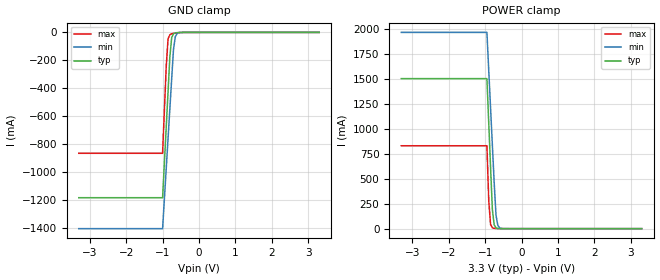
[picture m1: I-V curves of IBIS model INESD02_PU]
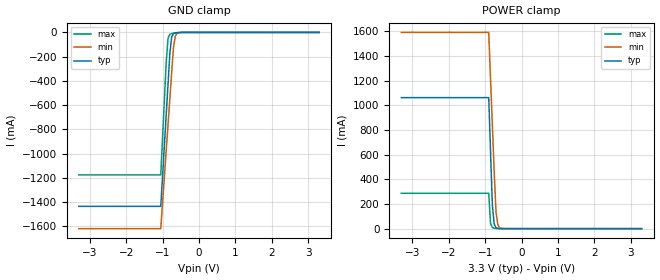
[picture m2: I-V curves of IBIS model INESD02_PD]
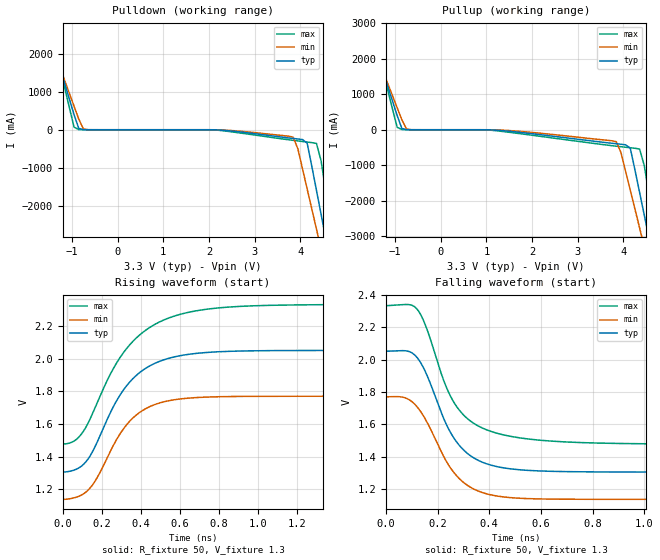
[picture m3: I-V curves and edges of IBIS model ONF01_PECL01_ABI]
|   This file is an IBIS representation of the   |
|   Integrated Devices Technology, Inc.   |
|   ICS843003I-01   |
|   FEMTOCLOCKS CRYSTAL-TO-3.3V/2.5V LVPECL FREQUENCY SYNTHESIZER   |
[IBIS Ver]   4.1
[File name]   843003i_01_3v3.ibs
[File Rev]   1.0
[Date]   24 Dec 2008 | Last modified
|   24 Dec 2008 | Generated
[Source]   Originated at Integrated Devices Technology, Inc.
[Disclaimer]
IDT hereby grants the user of this IBIS model a non-exclusive,
nontransferable license to use this IBIS model under the following terms.
Before using this IBIS model, the user should read this license.
If the user does not accept these terms,  the IBIS model should be
returned to IDT within 30 days.
   The user is granted this license only to use the IBIS model and
is not granted rights to sell, load, rent, lease or license the IBIS
model in whole or in part, or in modified form to anyone other than
user. User may modify the IBIS model to suit its specific
applications but rights to derivative works and such modifications
shall belong to IDT.
   This IBIS model is provided on an "AS IS" basis and IDT makes
absolutely no warranty with respect to the information contained
herein. IDT DISCLAIMS AND CUSTOMER WAIVES ALL WARRANTIES, EXPRESS
OR IMPLIED, INCLUDING WARRANTIES OF MERCHANTABILITY OR FITNESS FOR
A PARTICULAR PURPOSE. The entire risk as to quality and performance
is with the Customer. ACCORDINGLY, IN NO EVENT SHALL THE COMPANY BE
LIABLE FOR ANY DAMAGES, WHETHER IN CONTRACT OR TORT,INCLUDING ANY
LOST PROFITS OR OTHER INCIDENTAL, CONSEQUENTIAL, EXEMPLARY, OR
PUNITIVE DAMAGES ARISING OUT OF THE USE OR APPLICATION OF THE IBIS
model provided in this package. Further, IDT reserves the right to
make changes without notice to any product herein to improve
reliability, function, or design. IDT does not convey any license
under patent rights or any other intellectual property rights,
including those of third parties.
   IDT is not obligated to provide maintenance or support
for the licensed IBIS model.
[Copyright]   Copyright 2004 byIntegrated Devices Technology, Inc.
[Component]   ICS843003I-01
[Manufacturer] Integrated Devices Technology, Inc.
[Package]
|TSSOP 24 Lead
|   typ   min   max
R_pkg   60.65m   52.4m   68.9m
L_pkg   1.989nH   1.431nH   2.547nH
C_pkg   0.314pF   0.254pF   0.374pF
[Pin]   signal_name   model_name   R_pin   L_pin   C_pin
1   DIV_SELB0   INESD02_PU   68.9m   2.547n   0.374p
2   VCO_SEL   INESD02_PU   65.6m   2.323n   0.350p
3   MR   INESD02_PD   62.3m   2.100n   0.326p
4   VCCO_A   POWER   59.0m   1.877n   0.302p
5   QA0   ONF01_PECL01_ABI   55.7m   1.654n   0.278p
6   nQA0   ONF01_PECL01_ABI   52.4m   1.431n   0.254p
7   OEB   INESD02_PU_PECL   52.4m   1.431n   0.254p
8   OEA   INESD02_PU_PECL   55.7m   1.654n   0.278p
9   FB_DIV   INESD02_PD   59.0m   1.877n   0.302p
10   VCCA   POWER   62.3m   2.100n   0.326p
11   VCC   POWER   65.6m   2.323n   0.350p
12   DIV_SELA0   INESD02_PU   68.9m   2.547n   0.374p
13   DIV_SELA1   INESD02_PU   68.9m   2.547n   0.374p
14   VEE   GND   65.6m   2.323n   0.350p
15   XTAL_OUT   NC   62.3m   2.100n   0.326p
16   XTAL_IN   NC   59.0m   1.877n   0.302p
17   REF_CLK   INESD02_PD_PECL   55.7m   1.654n   0.278p
18   XTAL_SEL   INESD02_PU   52.4m   1.431n   0.254p
19   nQB1   ONF01_PECL01_ABI   52.4m   1.431n   0.254p
20   QB1   ONF01_PECL01_ABI   55.7m   1.654n   0.278p
21   nQB0   ONF01_PECL01_ABI   59.0m   1.877n   0.302p
22   QB0   ONF01_PECL01_ABI   62.3m   2.100n   0.326p
23   VCCO_B   POWER   65.6m   2.323n   0.350p
24   DIV_SELB1   INESD02_PU   68.9m   2.547n   0.374p
[Diff Pin]  inv_pin  vdiff tdelay_typ tdelay_min  tdelay_max
5   6   NA   0   0   0
20   19   NA   0   0   0
23   22   NA   0   0   0
| Models and submodels in the file (5): INESD02_PU (Input), INESD02_PD (Input), ONF01_PECL01_ABI (Output_ECL), INESD02_PU_PECL (Input), INESD02_PD_PECL (Input)
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[Model]   INESD02_PU
Model_type   Input
Polarity   Non-Inverting
Vinl = 0.80V
Vinh = 2.0V
|   typ   min   max
C_comp   2pF   1.5pF   2.5pF
|   typ   min   max
[Voltage range]  3.3V   3.15V   3.45V
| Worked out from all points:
|   GND clamp passes 1 mA (typ) near -0.56 V on its own axis
|   POWER clamp passes 1 mA (typ) near -0.61 V on its own axis
[GND_clamp]
|Voltage   I(typ)   I(min)   I(max)
-3.3V     -1.184A    -1.405A    -865.6mA
-1V       -1.184A    -1.405A    -865.6mA
-900mV    -678.5mA   -975.1mA   -244.1mA
-850mV    -426.2mA   -760.2mA   -46.92mA
-800mV    -174mA     -545.4mA   -16.17mA
-750mV    -37.03mA   -330.8mA   -9.981mA
-700mV    -9.767mA   -120.3mA   -7.122mA
-650mV    -3.616mA   -29.78mA   -4.922mA
-600mV    -1.7mA     -7.594mA   -3.115mA
-400mV    -123.9uA   -126uA     -173.9uA
3.3V      1.866nA    3.949uA    0A
[POWER_clamp]
|Voltage   I(typ)   I(min)   I(max)
-3.3V     1.506A     1.97A      832.1mA
-950mV    1.506A     1.97A      832.1mA
-900mV    1.063A     1.592A     287.2mA
-850mV    620.4mA    1.215A     41.77mA
-800mV    191.5mA    837.4mA    8.692mA
-750mV    37.69mA    460.1mA    3.262mA
-700mV    8.032mA    133.8mA    1.662mA
-650mV    2.005mA    32.58mA    840.1uA
-600mV    607uA      8.009mA    378.6uA
-450mV    33.11uA    139.8uA    23.88uA
3.3V      -71.13uA   -77.46uA   -62.11uA
[Model]   INESD02_PD
Model_type   Input
Polarity   Non-Inverting
Vinl = 0.80V
Vinh = 2.0V
|   typ   min   max
C_comp   2pF   1.5pF   2.5pF
|   typ   min   max
[Voltage range]  3.3V   3.15V   3.45V
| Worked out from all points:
|   GND clamp passes 1 mA (typ) near -0.56 V on its own axis
|   POWER clamp passes 1 mA (typ) near -0.61 V on its own axis
[GND_clamp]
|Voltage   I(typ)   I(min)   I(max)
-3.3V     -1.436A    -1.62A     -1.176A
-1.05V    -1.436A    -1.62A     -1.176A
-900mV    -678.5mA   -975.1mA   -244mA
-850mV    -426.1mA   -760.1mA   -46.85mA
-800mV    -173.9mA   -545.4mA   -16.11mA
-750mV    -36.96mA   -330.7mA   -9.916mA
-700mV    -9.696mA   -120.2mA   -7.056mA
-650mV    -3.545mA   -29.7mA    -4.857mA
-600mV    -1.629mA   -7.52mA    -3.049mA
-400mV    -52.81uA   -52.52uA   -108.7uA
3.3V      71.13uA    77.43uA    62.11uA
[POWER_clamp]
|Voltage   I(typ)   I(min)   I(max)
-3.3V     1.063A     1.593A     287.3mA
-900mV    1.063A     1.593A     287.3mA
-850mV    620.5mA    1.215A     41.84mA
-800mV    191.6mA    837.5mA    8.757mA
-750mV    37.76mA    460.2mA    3.328mA
-700mV    8.104mA    133.8mA    1.728mA
-650mV    2.076mA    32.66mA    905.3uA
-600mV    678.1uA    8.083mA    443.8uA
-450mV    104.2uA    213.3uA    89.09uA
3.3V      -3.041nA   -3.986uA   0A
[Model]   ONF01_PECL01_ABI
Model_type  Output_ECL
Polarity   Non-Inverting
Vmeas = 1.63
Rref = 50
Cref = 0
Vref = 1.3
|Variable  typ   min   max
C_comp   2p   1.5p   2.5p
[Voltage Range]   3.3   3.135   3.465
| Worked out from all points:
|   rising waveform, R_fixture 50, V_fixture 1.3: 20-80 % time 218ps typ, 193ps min, 263ps max; typ from 1.31 V to 2.05 V
|   falling waveform, R_fixture 50, V_fixture 1.3: 20-80 % time 134ps typ, 136ps min, 142ps max; typ from 2.05 V to 1.31 V
| Open source, no load
|  Voltage   I(typ)   I(min)   I(max)
[Pulldown]
-3.3V     9.786A     8.425A     12.06A
-1.667V   3.247A     2.986A     3.704A
-1.463V   2.432A     2.308A     2.661A
-952.6mV  398mA      618.5mA    68.87mA
-850.5mV  36.63mA    281.6mA    4.032mA
3.844V    -229.1mA   -195.7mA   -279.4mA
4.151V    -352.7mA   -1.559A    -324.9mA
4.355V    -1.599A    -2.62A     -360.9mA
4.559V    -2.871A    -3.681A    -1.635A
4.661V    -3.508A    -4.211A    -2.446A
4.763V    -4.144A    -4.742A    -3.257A
6.6V      -15.69A    -14.35A    -17.99A
[Pullup]
-3.3V     9.786A     8.425A     12.06A
-1.565V   2.839A     2.647A     3.182A
-952.6mV  398mA      618.5mA    68.87mA
-850.5mV  36.63mA    281.6mA    4.032mA
-646.4mV  229.3uA    964.8uA    177.5uA
3.844V    -394.4mA   -337mA     -463.1mA
4.151V    -517.8mA   -1.701A    -507.4mA
4.355V    -1.764A    -2.763A    -542.7mA
4.559V    -3.036A    -3.825A    -1.816A
4.661V    -3.672A    -4.355A    -2.626A
4.763V    -4.308A    -4.886A    -3.437A
6.6V      -15.79A    -14.46A    -18.06A
[Ramp]
|   typ   min   max
dV/dt_r   0.596/0.354n   0.506/0.311n   0.684/0.427n
dV/dt_f   0.599/0.219n   0.507/0.219n   0.690/0.252n
R_load =   50.0000
[Rising Waveform]
R_fixture = 50
V_fixture = 1.3   | VCC_typ - 2V
V_fixture_max = 1.465   | VCC_max - 2V
V_fixture_min = 1.135   | VCC_min - 2V
C_fixture = 0.0p
| Time   typ   min   max
0s        1.306V     1.138V     1.478V
67.2ps    1.321V     1.15V      1.503V
126ps     1.379V     1.19V      1.597V
176.4ps   1.489V     1.271V     1.731V
247.8ps   1.679V     1.442V     1.915V
338.1ps   1.85V      1.61V      2.079V
430.5ps   1.946V     1.698V     2.18V
554.4ps   2.007V     1.745V     2.255V
936.6ps   2.049V     1.77V      2.324V
1.999ns   2.052V     1.771V     2.333V
[Falling Waveform]
R_fixture = 50
V_fixture = 1.3   | VCC_typ - 2V
V_fixture_max = 1.465   | VCC_max - 2V
V_fixture_min = 1.135   | VCC_min - 2V
C_fixture = 0.0p
| Time   typ   min   max
0s        2.052V     1.771V     2.334V
73.5ps    2.055V     1.765V     2.34V
119.7ps   2.015V     1.711V     2.314V
151.2ps   1.932V     1.637V     2.221V
224.7ps   1.633V     1.399V     1.868V
268.8ps   1.503V     1.293V     1.723V
336ps     1.398V     1.205V     1.611V
434.7ps   1.338V     1.157V     1.544V
806.4ps   1.307V     1.138V     1.486V
1.999ns   1.306V     1.138V     1.478V
